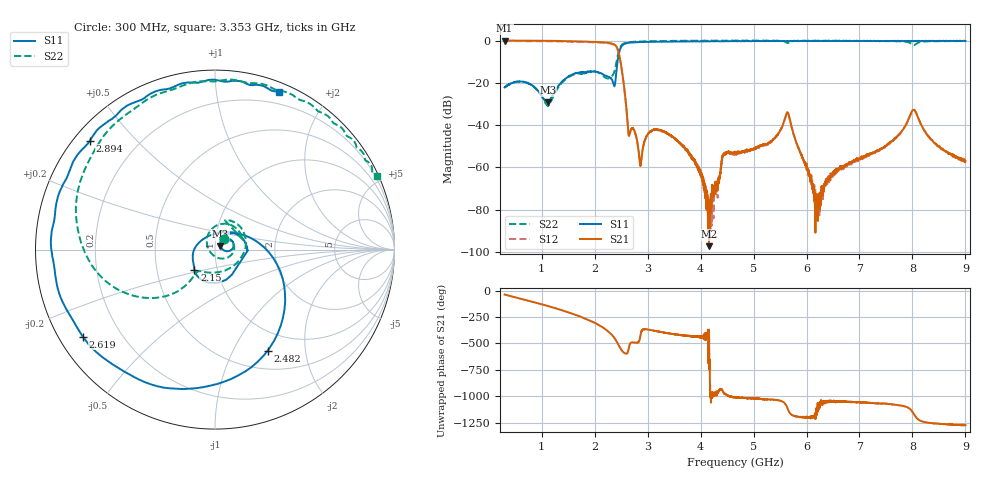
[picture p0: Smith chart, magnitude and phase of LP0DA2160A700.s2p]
!Agilent Technologies,E8358A,US41080443,A.07.50.56
!Agilent E8358A: A.07.50.56
!Date: Friday, August 05, 2016 08:34:12
!Correction: S11(Full 2 Port(1,2))
!S21(Full 2 Port(1,2))
!S12(Full 2 Port(1,2))
!S22(Full 2 Port(1,2))
!S2P File: Measurements: S11, S21, S12, S22:Log Frequency Sweep
# Hz S  dB  R 50
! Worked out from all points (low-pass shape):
!   6401 points, 300 MHz to 9 GHz, reference 50 ohm
!   highest |S21| = 0.06 dB at 300.3 MHz (marker M1); lowest = -97.2 dB at 4.158 GHz (marker M2)
!   |S21| within 3 dB of the highest: start of sweep to 2.413 GHz
!   lowest |S11| = -29.1 dB at 1.12 GHz (marker M3), VSWR 1.07, Z = 53.1 + j1.88 ohm
!   |S11| at or under -10 dB: start of sweep to 2.432 GHz
!   |S22| runs from -30.8 to 0.1 dB; largest |S21 - S12| = 0.028
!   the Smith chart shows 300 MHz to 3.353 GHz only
!   S11 on the Smith chart (normalised r, x): 300 MHz: 1.09, +0.14; 2.15 GHz: 0.77, -0.18; 2.482 GHz: 0.73, -1.38; 2.619 GHz: 0.07, -0.30; 2.894 GHz: 0.05, +0.37; 3.353 GHz: 0.08, +1.48
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3e8  -22.12 52.0  0.06 -38.3  -0.18 -38.1  -22.15 48.1
3.00319e8  -22.11 52.0  0.06 -38.3  -0.18 -38.2  -22.15 48.1
7.187151e8  -19.83 6.3  -0.05 -91.9  -0.27 -91.7  -19.93 -10.6
1.119552e9  -29.12 30.3  -0.09 -147.1  -0.31 -147.0  -30.73 -141.7
1.75044e9  -14.94 2.7  -0.43 108.8  -0.66 108.9  -15.54 33.2
2.15014e9  -15.79 -135.1  -0.77 11.6  -1.01 11.8  -16.47 -19.8
2.353438e9  -20.30 155.3  -1.62 -76.2  -1.85 -76.0  -15.91 -128.8
2.481892e9  -3.93 -62.6  -8.96 176.0  -9.19 175.8  -3.15 -173.4
2.618748e9  -1.09 -146.6  -37.72 128.6  -38.03 128.9  -0.89 121.1
2.893904e9  -0.69 138.9  -53.72 -17.1  -53.89 -14.5  -0.35 66.8
3.201372e9  -0.57 86.9  -42.10 -28.2  -42.41 -28.4  -0.21 35.3
3.352863e9  -0.46 68.0  -43.62 -41.8  -43.76 -41.6  -0.10 24.4
3.876361e9  -0.31 20.5  -56.34 -75.2  -56.46 -70.3  0.00 -1.2
4.158051e9  -0.31 3.1  -97.22 -161.7  -82.71 -28.5  -0.05 -10.6
4.462582e9  -0.23 -10.0  -53.25 99.6  -53.68 104.8  0.06 -18.1
4.651453e9  -0.20 -16.6  -53.17 72.5  -53.41 69.7  0.06 -21.9
5.638172e9  -0.13 -40.6  -33.87 -29.7  -34.11 -29.8  -1.09 -40.0
6.102778e9  -0.11 -48.8  -66.19 -128.0  -67.71 -117.7  0.01 -47.1
6.240526e9  -0.15 -51.1  -77.46 15.8  -78.53 0.9  -0.04 -50.2
7.552286e9  -0.19 -72.9  -48.59 6.1  -48.81 5.8  -0.23 -89.0
8.03678e9  -0.17 -79.9  -32.74 -97.7  -32.99 -97.7  -2.11 -102.1
9e9  -0.14 -93.5  -57.00 165.6  -56.67 167.1  -0.19 -132.8
